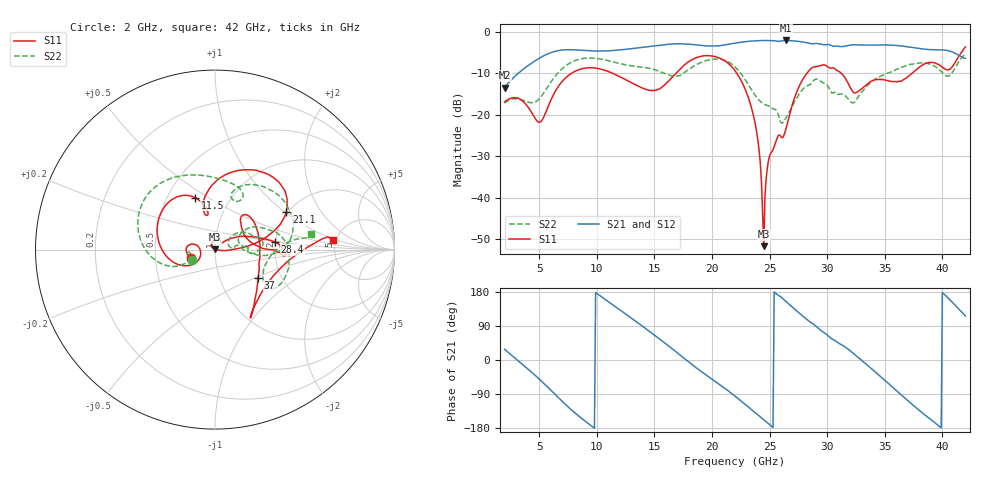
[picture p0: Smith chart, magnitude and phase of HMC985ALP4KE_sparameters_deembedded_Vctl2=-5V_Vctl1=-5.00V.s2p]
!s2p File: Measurements: S11, S21, S12, S22
# GHz S dB R 50.0
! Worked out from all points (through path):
!   401 points, 2 GHz to 42 GHz, reference 50 ohm
!   highest |S21| = -2.06 dB at 26.4 GHz (marker M1); lowest = -13.4 dB at 2 GHz (marker M2)
!   lowest |S11| = -51.7 dB at 24.5 GHz (marker M3), VSWR 1.01, Z = 49.9 + j0.237 ohm
!   |S11| at or under -10 dB: start of sweep to 7.81 GHz; 22.16 GHz to 28.24 GHz (6.081 GHz wide, 24.1 % of centre); 31.23 GHz to 37.36 GHz (6.136 GHz wide, 17.9 % of centre)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
!   |S22| runs from -22.0 to -5.4 dB; largest |S21 - S12| = 0.0011
!   S11 on the Smith chart (normalised r, x): 2 GHz: 0.76, -0.07; 11.5 GHz: 0.68, +0.44; 21.1 GHz: 1.96, +1.03; 28.4 GHz: 1.99, +0.19; 37 GHz: 1.53, -0.52; 42 GHz: 4.69, +0.86
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2  -16.89 -161.7  -13.43 28.3  -13.43 28.3  -17.19 -155.5
5  -21.82 -172.3  -6.37 -50.1  -6.37 -50.1  -16.18 -159.6
6.3  -14.84 -150.2  -4.76 -88.3  -4.76 -88.3  -11.03 -161.4
8.7  -8.91 150.5  -4.44 -154.5  -4.44 -154.5  -6.46 151.4
11.5  -10.16 111.2  -4.47 143.3  -4.47 143.3  -7.31 105.2
13.6  -13.11 101.2  -3.86 97.3  -3.86 97.3  -8.40 75.8
15.4  -13.82 105.8  -3.26 56.7  -3.26 56.7  -9.49 62.1
17.9  -7.34 80.5  -2.95 -3.3  -2.95 -3.2  -9.21 72.2
21.1  -6.96 27.8  -3.15 -74.1  -3.15 -74.1  -6.86 16.3
22  -9.34 17.3  -2.72 -95.3  -2.72 -95.2  -8.44 0.8
23.6  -20.18 0.1  -2.18 -134.9  -2.18 -134.9  -14.70 -4.3
24  -26.51 -7.0  -2.11 -144.9  -2.12 -144.9  -16.21 1.1
24.5  -51.75 113.3  -2.08 -157.6  -2.08 -157.5  -17.39 8.0
25  -29.94 133.5  -2.10 -170.3  -2.11 -170.3  -17.97 10.8
26.4  -23.65 41.8  -2.06 155.0  -2.06 155.1  -20.89 33.2
28.4  -9.45 7.2  -2.72 103.1  -2.72 103.1  -12.87 18.8
28.7  -8.62 2.3  -2.86 96.8  -2.86 96.9  -12.19 16.8
32.5  -14.68 31.4  -3.10 11.4  -3.10 11.4  -16.53 27.5
35.4  -11.84 19.5  -3.17 -64.1  -3.17 -64.0  -9.83 19.6
37  -10.85 -33.1  -3.59 -107.2  -3.59 -107.2  -8.03 5.4
39.8  -8.11 -57.2  -4.31 -176.6  -4.31 -176.5  -9.28 -35.3
42  -3.63 4.5  -6.34 115.8  -6.34 115.8  -5.37 9.0
